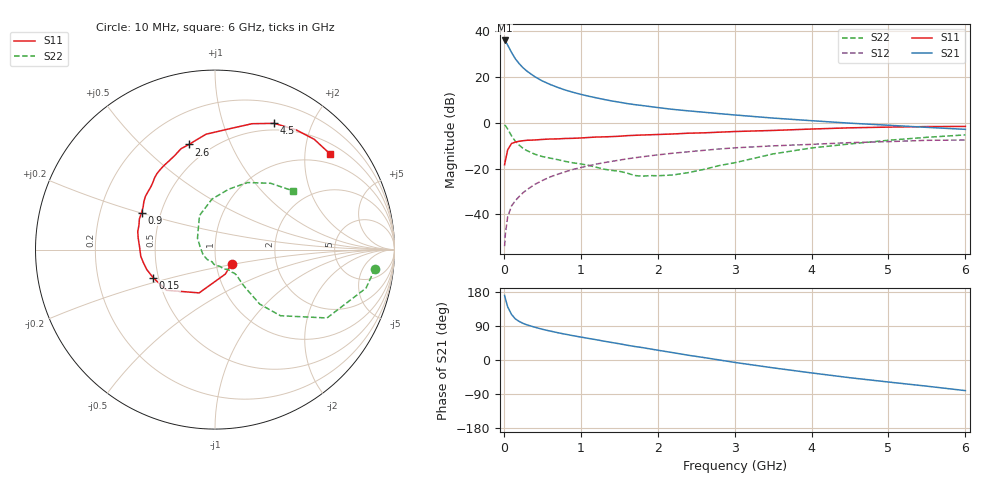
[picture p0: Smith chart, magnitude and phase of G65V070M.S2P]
! SIEMENS Small Signal Semiconductors
! BFG193
! Si NPN RF Bipolar Junction Transistor in SOT223
! VCE = 5 V  IC = 70 mA
! Common Emitter S-Parameters:  August  1996
# GHz  S  MA  R  50
!  f  S11  S21  S12  S22
! GHz  MAG  ANG  MAG  ANG  MAG  ANG  MAG  ANG
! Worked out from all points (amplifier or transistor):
!   36 points, 10 MHz to 6 GHz, reference 50 ohm
!   highest |S21| = 36.0 dB at 10 MHz (marker M1)
!   |S21| within 3 dB of that: start of sweep to 65.02 MHz
!   unconditionally stable (mu >= 1): 361 MHz to 2.331 GHz
!   at 250 MHz: K = 0.95, MSG = 27.3 dB, |S12| = -30.6 dB
!   at 1.4 GHz: K = 1.05, MAG = 11.9 dB, |S12| = -16.9 dB
!   at 6 GHz: K = 0.90, MSG = 2.3 dB, |S12| = -7.5 dB
!   S11 on the Smith chart (normalised r, x): 10 MHz: 1.19, -0.19; 150 MHz: 0.47, -0.17; 900 MHz: 0.39, +0.20; 2.6 GHz: 0.38, +0.71; 4.5 GHz: 0.42, +1.49; 6 GHz: 0.74, +2.59
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0.01  0.1209 -40.2  63.41 170.3  0.002 82.6  0.8975 -6.8
0.02  0.1482 -67.2  61.01 161.9  0.0037 81.0  0.8684 -14.3
0.05  0.2568 -110.1  50.17 140.2  0.0088 71.6  0.731 -31.4
0.1  0.3528 -140.0  34.64 120.2  0.0152 69.0  0.5184 -45.3
0.15  0.3781 -155.5  25.09 108.3  0.0198 68.6  0.393 -50.6
0.2  0.3959 -163.6  19.67 101.8  0.0245 70.6  0.3243 -51.0
0.25  0.4058 -169.8  16 96.6  0.0296 70.5  0.2749 -51.4
0.3  0.4152 -174.8  13.53 92.7  0.0344 71.2  0.247 -51.5
0.4  0.4209 177.7  10.27 86.7  0.0447 71.0  0.2066 -50.5
0.5  0.4331 171.3  8.247 81.1  0.0546 69.9  0.183 -49.9
0.6  0.442 166.8  6.929 76.5  0.0652 69.0  0.1693 -50.9
0.7  0.4451 162.1  5.957 72.1  0.0749 67.5  0.1564 -53.2
0.9  0.4582 153.2  4.65 64.2  0.0955 63.5  0.1333 -56.4
1.1  0.4777 146.1  3.828 57.0  0.1147 60.2  0.1175 -65.9
1.3  0.4926 139.7  3.25 49.8  0.1343 55.9  0.0969 -74.1
1.6  0.5235 129.9  2.644 39.1  0.1628 49.0  0.0797 -95.9
2.2  0.5703 113.1  1.967 19.3  0.2165 35.4  0.0723 -159.9
2.6  0.6036 103.9  1.706 6.5  0.2499 26.6  0.0956 158.3
3.5  0.681 82.5  1.27 -20.7  0.3132 4.0  0.2088 114.4
4.5  0.7774 64.8  0.982 -46.8  0.3683 -16.1  0.3452 77.2
5.5  0.8267 48.0  0.796 -69.1  0.4142 -39.6  0.4823 50.0
6  0.8338 39.6  0.72 -80.8  0.4198 -53.1  0.5441 37.0
